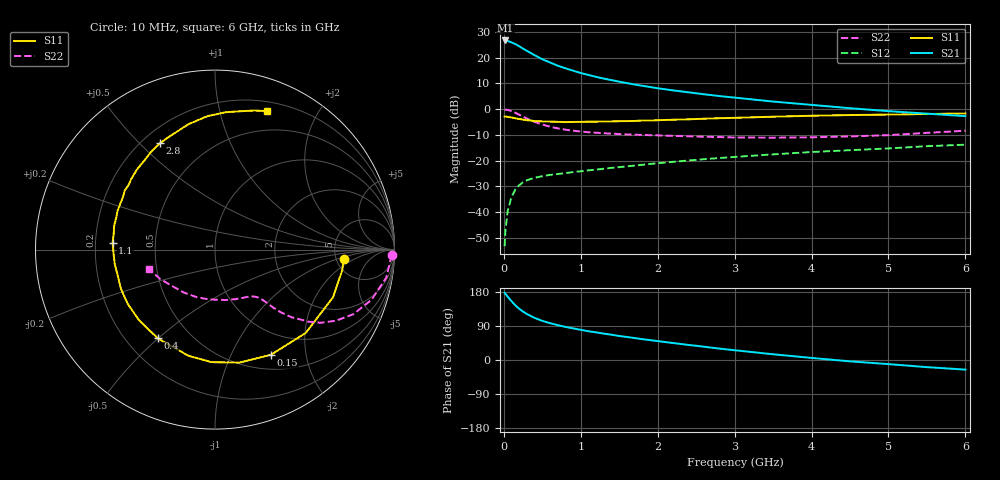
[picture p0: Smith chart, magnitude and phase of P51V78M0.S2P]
! SIEMENS Small Signal Semiconductors
! BFP183
! Si NPN RF Bipolar Junction Transistor in SOT143
! VCE = 1.75 V  IC = 8 mA
! Common Emitter S-Parameters:  March  1996
# GHz  S  MA  R  50
!  f  S11  S21  S12  S22
! GHz  MAG  ANG  MAG  ANG  MAG  ANG  MAG  ANG
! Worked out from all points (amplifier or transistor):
!   36 points, 10 MHz to 6 GHz, reference 50 ohm
!   highest |S21| = 26.6 dB at 20 MHz (marker M1)
!   |S21| within 3 dB of that: start of sweep to 240.3 MHz
!   unconditionally stable (mu >= 1): 1.232 GHz to 5.636 GHz
!   at 250 MHz: K = 0.29, MSG = 25.9 dB, |S12| = -28.3 dB
!   at 1.4 GHz: K = 1.05, MAG = 15.6 dB, |S12| = -22.8 dB
!   at 6 GHz: K = 0.96, MSG = 5.5 dB, |S12| = -13.8 dB
!   S11 on the Smith chart (normalised r, x): 10 MHz: 5.79, -1.32; 150 MHz: 0.68, -1.43; 400 MHz: 0.33, -0.50; 1.1 GHz: 0.27, +0.03; 2.8 GHz: 0.27, +0.58; 6 GHz: 0.29, +1.40
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0.01  0.7181 -4.4  21.34 177.6  0.0022 86.8  0.9863 -1.8
0.02  0.7186 -9.1  21.48 175.2  0.0043 89.9  0.9783 -3.7
0.05  0.7089 -22.1  21.05 167.0  0.0106 81.9  0.9671 -9.3
0.1  0.6865 -42.6  19.69 155.1  0.0198 70.2  0.9155 -17.8
0.15  0.6636 -62.0  18.27 144.2  0.0278 61.7  0.851 -25.0
0.2  0.6442 -77.9  16.59 135.2  0.0336 56.5  0.7812 -30.5
0.25  0.6273 -91.8  14.89 127.6  0.0383 51.1  0.716 -34.7
0.3  0.6097 -104.1  13.52 121.4  0.0418 47.7  0.6563 -37.7
0.4  0.5884 -122.8  11.12 111.0  0.0467 42.8  0.5653 -41.6
0.5  0.5777 -137.1  9.285 103.3  0.05 39.7  0.503 -43.7
0.6  0.5727 -148.3  8.04 97.2  0.0531 38.1  0.4575 -44.9
0.7  0.5678 -157.4  6.969 92.0  0.0552 37.5  0.4235 -45.6
0.9  0.5643 -171.8  5.573 83.5  0.0601 37.6  0.3814 -46.8
1.1  0.5717 176.1  4.606 75.9  0.0651 37.8  0.3564 -48.2
1.5  0.584 158.5  3.408 63.4  0.075 39.0  0.3288 -52.4
1.8  0.6014 146.8  2.84 55.0  0.0833 39.5  0.3159 -56.9
2.2  0.6234 134.2  2.312 44.7  0.0951 39.0  0.3029 -64.1
2.8  0.6672 117.4  1.796 30.1  0.1127 36.6  0.2878 -77.5
3.5  0.7135 102.1  1.404 15.1  0.1328 33.3  0.2797 -96.0
4.5  0.7675 85.6  1.043 -3.6  0.1599 26.6  0.2959 -126.2
5.5  0.8047 74.3  0.818 -18.8  0.1912 20.2  0.3469 -151.9
6  0.8244 69.4  0.732 -25.4  0.2046 15.8  0.3817 -163.2
